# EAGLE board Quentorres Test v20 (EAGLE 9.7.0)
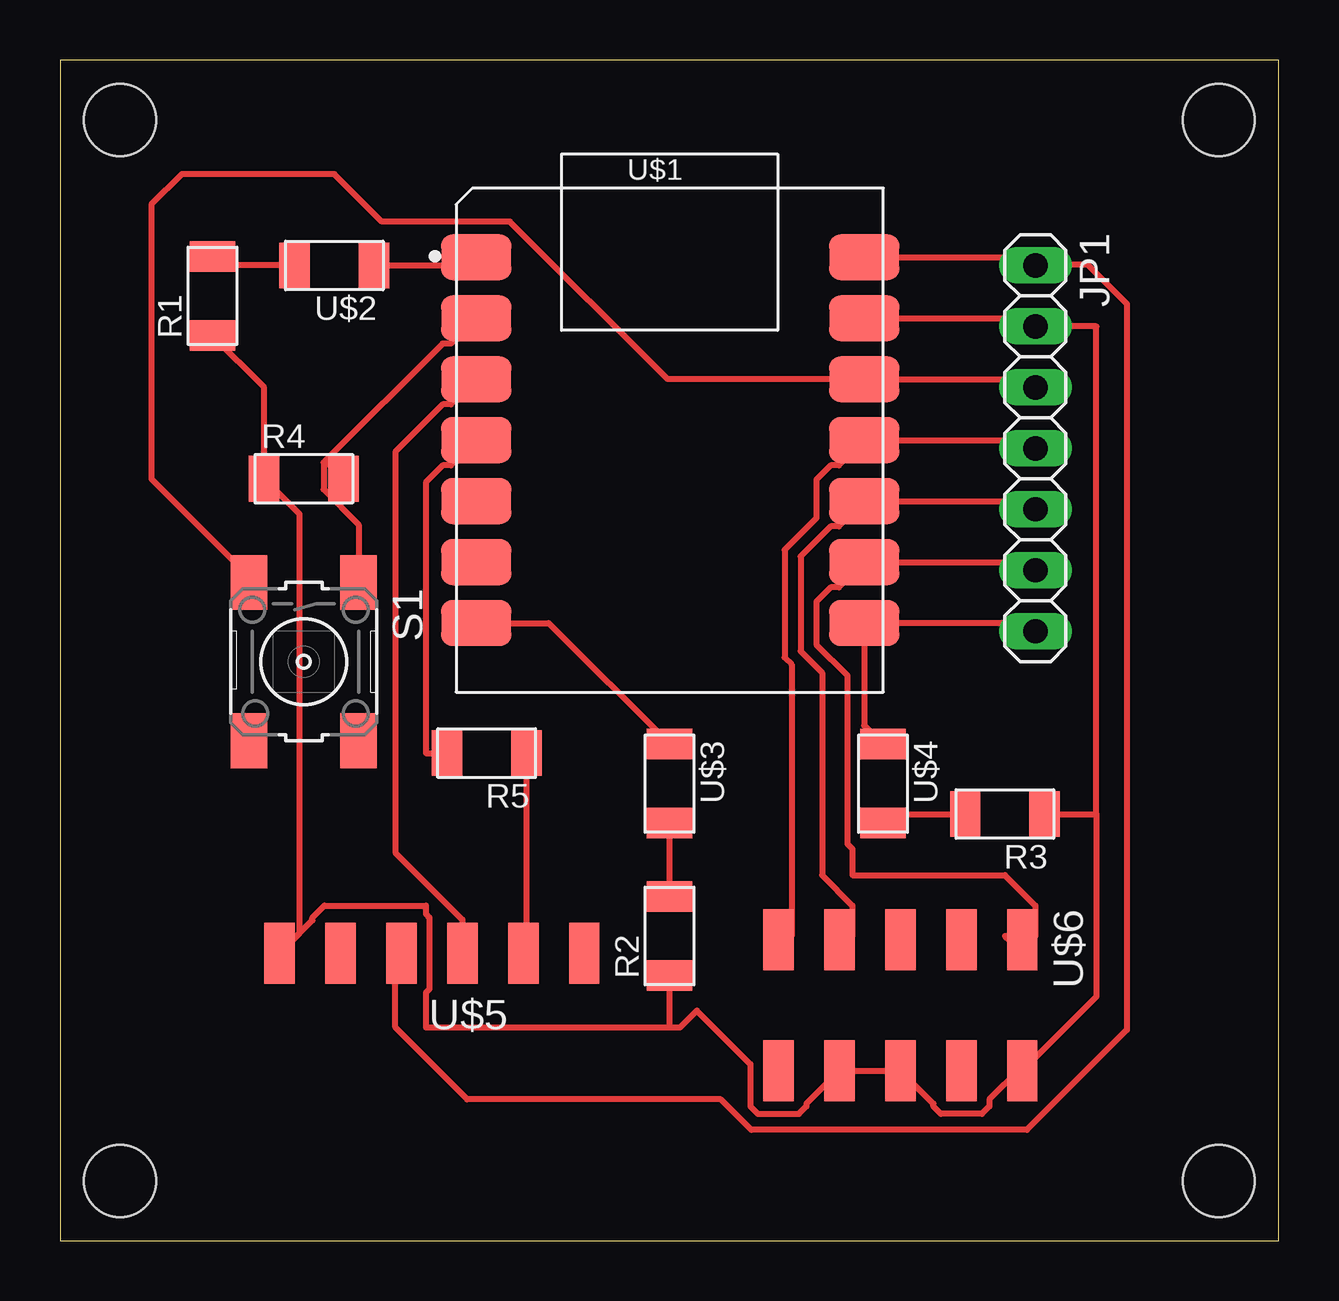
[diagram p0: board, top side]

Size 50.78 x 49.2 mm. Coordinates in mm from the lower left corner, seen from the top.
Outline: 0,49.2 0,0 50.78,0 50.78,49.2 0,49.2
Copper layers (1*16): Top 0.035mm / dielectric 1.5mm / Bottom 0.035mm
Design rules "fab.dru": minimum track width 10mil, minimum drill 32mil, track to track 16mil, track to pad 16mil, pad to pad 16mil, via to via 16mil, smd to smd 6mil, copper to edge 16mil, drill to drill 16mil, minimum pad ring 10mil, minimum via ring 8mil, stop-mask expansion 4mil, vias tented up to drill 0mil, thermal gap 16mil
Holes 3 mm at 2.5,46.7 48.28,46.7 2.5,2.5 48.28,2.5

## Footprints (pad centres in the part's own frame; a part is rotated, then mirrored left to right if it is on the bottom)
1X07 = drill 1.016 long: 1 -7.62,0; 2 -5.08,0; 3 -2.54,0; 4 0,0; 5 2.54,0; 6 5.08,0; 7 7.62,0
R1206FAB = smd 1.27 x 1.905: 1 -1.651,0; 2 1.651,0
6MM_SWITCH = smd 2.286 x 1.524: 1 -3.302,2.286; 2 3.302,2.286; 3 -3.302,-2.286; 4 3.302,-2.286
XIAO_RP2040_TAPED = smd 2.921 x 1.905: 1 0.835,18.12; 2 0.835,15.58; 3 0.835,13.04; 4 0.835,10.5; 5 0.835,7.96; 6 0.835,5.42; 7 0.835,2.88; 8 17,2.88; 9 17,5.42; 10 17,7.96; 11 17,10.5; 12 17,13.04; 13 17,15.58; 14 17,18.12
LED1206FAB = smd 1.27 x 1.905: 1 -1.651,0; 2 1.651,0
1X06SMD = smd 2.54 x 1.27: 1 0,6.35; 2 0,3.81; 3 0,1.27; 4 0,-1.27; 5 0,-3.81; 6 0,-6.35
2X05SMD = smd 2.54 x 1.27: 1 -2.54,2.54; 2 2.92,2.54; 3 -2.54,0; 4 2.92,0; 5 -2.54,-2.54; 6 2.92,-2.54; 7 -2.54,-5.08; 8 2.92,-5.08; 9 -2.54,-7.62; 10 2.92,-7.62

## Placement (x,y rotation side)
JP1  PINHD-1X7  [1X07]  40.64,33.02 270 top
R1  1k  [R1206FAB]  6.35,39.37 90 top
R2  1k  [R1206FAB]  25.4,12.7 90 top
R3  1k  [R1206FAB]  39.37,17.78 180 top
R4  470  [R1206FAB]  10.16,31.75 0 top
R5  1k  [R1206FAB]  17.78,20.32 180 top
S1  [6MM_SWITCH]  10.16,24.13 270 top
U$1  XIAO_RP2040  [XIAO_RP2040_TAPED]  16.51,22.86 0 top
U$2  LEDFAB1206  [LED1206FAB]  11.43,40.64 180 top
U$3  LEDFAB1206  [LED1206FAB]  25.4,19.05 270 top
U$4  LEDFAB1206  [LED1206FAB]  34.29,19.05 270 top
U$5  CONN_06_FTDI-SMD-HEADER  [1X06SMD]  15.49,11.98 90 top
U$6  CONN_05X2-PINHEAD-SMD  [2X05SMD]  37.55,10.01 270 top

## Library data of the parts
JP1 = Connector; CATEGORY: Headers; DESCRIPTION: Header-Straight-7 Position; PACKAGE_TYPE: THT; PITCH: 0.100" (2.54mm); SUBCATEGORY: Headers-Male Pins; TYPE: Board to Board or Cable-Unshrouded-Through Hole-Straight
R1-R5 S1 U$1-U$6 = fab

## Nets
3V3: JP1.3 S1.3 U$1.12
5V0: JP1.1 U$1.14 U$5.3
GND: JP1.2 R1.1 R2.1 R3.1 R4.1 U$1.13 U$5.1 U$6.2 U$6.6 U$6.8
N$1: R3.2 U$4.2
N$2: R2.2 U$3.2
N$3: R1.2 U$2.2
N$4: U$1.1 U$2.1
N$5: U$1.7 U$3.1
N$6: JP1.7 U$1.8 U$4.1
N$7: R4.2 S1.1 U$1.2
N$8: JP1.4 U$1.11 U$6.9
N$9: JP1.5 U$1.10 U$6.7
N$10: JP1.6 U$1.9 U$6.1
N$11: U$5.2
N$12: U$1.3 U$5.4
N$13: R5.2 U$1.4
N$14: R5.1 U$5.5
N$16: U$5.6

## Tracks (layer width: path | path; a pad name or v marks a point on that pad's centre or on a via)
3V3
  Top 0.254: JP1.3 40.3,35.9 U$1.12 25.31,35.9 18.75,42.47 13.41,42.47 11.43,44.45 5.08,44.45 3.81,43.18 3.81,31.75 7.87,27.69 S1.3
5V0
  Top 0.254: U$1.14 40.3,40.98 JP1.1 40.67,40.67 42.82,40.67 44.45,39.03 44.45,8.78 40.29,4.62 28.8,4.62 27.53,5.89 16.97,5.89 13.97,8.89 13.97,11.72 U$5.3
GND
  Top 0.254: U$1.13 40.3,38.44 JP1.2 43.18,38.1 43.18,17.78 | R1.1 8.51,35.56 R4.1 9.97,30.29 9.97,12.8 U$5.1 10.52,13.35 10.52,13.47 11.02,13.97 15.24,13.97 15.24,13.62 15.39,13.47 15.39,10.48 15.24,10.33 15.24,8.89 25.4,8.89 | 25.4,8.89 R2.1 | 25.4,8.89 25.84,8.89 26.54,9.59 28.77,7.36 28.77,5.6 29.08,5.28 30.79,5.28 31.1,5.6 31.1,5.72 U$6.8 U$6.6 36.39,5.72 36.39,5.6 36.7,5.28 38.41,5.28 38.72,5.6 38.72,5.89 40.01,7.18 U$6.2 43.18,10.17 43.18,17.78 | R3.1 43.18,17.78
N$1
  Top 0.254: U$4.2 34.67,17.78 R3.2
N$2
  Top 0.254: R2.2 U$3.2
N$3
  Top 0.254: U$2.2 6.73,40.64 R1.2
N$4
  Top 0.254: U$1.1 17,40.64 U$2.1
N$5
  Top 0.254: U$3.1 20.36,25.74 U$1.7
N$6
  Top 0.254: JP1.7 40.3,25.74 U$1.8 33.51,21.48 U$4.1
N$7
  Top 0.254: 11.06,32.5 R4.2 | S1.1 12.45,29.84 10.99,31.3 10.99,32.43 11.06,32.5 | U$1.2 16.29,37.39 15.94,37.39 11.06,32.5
N$8
  Top 0.254: JP1.4 40.3,33.36 U$1.11 32.46,32.31 32.11,32.31 31.52,31.71 31.52,30.11 30.2,28.79 30.2,24.3 30.48,24.01 30.48,12.7 30.33,12.55 U$6.9
N$9
  Top 0.254: JP1.5 40.3,30.82 U$1.10 32.46,29.77 32.11,29.77 30.86,28.51 30.86,24.57 31.75,23.68 31.75,15.24 33.02,13.97 33.02,12.7 32.87,12.55 U$6.7
N$10
  Top 0.254: JP1.6 40.3,28.28 U$1.9 32.46,27.23 32.11,27.23 31.52,26.63 31.52,24.85 32.8,23.56 32.8,16.54 33.02,16.33 33.02,15.24 39.37,15.24 40.64,13.97 40.64,12.7 39.37,12.7 39.52,12.55 U$6.1
N$12
  Top 0.254: U$5.4 16.76,13.38 13.97,16.17 13.97,32.87 15.94,34.85 16.29,34.85 U$1.3
N$13
  Top 0.254: U$1.4 16.29,32.31 15.94,32.31 15.24,31.6 15.24,20.32 R5.2
N$14
  Top 0.254: R5.1 19.43,13.08 19.05,12.7 19.05,12.23 U$5.5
